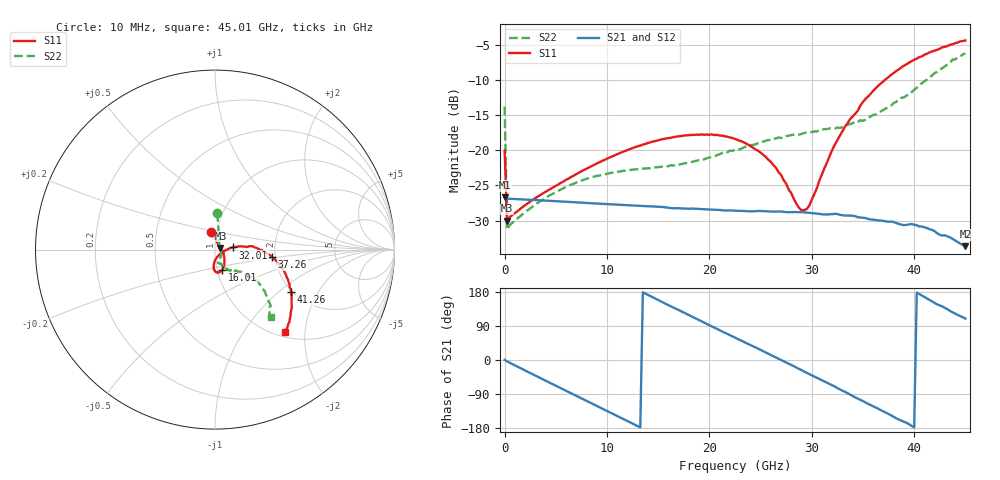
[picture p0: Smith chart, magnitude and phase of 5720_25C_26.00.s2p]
! Device:  ADRF5720
! Description: 0.5dB LSB GaAs MMIC 6-bit Digital Attenuator
! Frequency:  0.000009 -  40 GHz
! Ports:
!	RF1	= Port 1
!	RF2	= Port 2
! Vdd:  3.3 Volt
! Vss:  -3.3 Volt
! Control:  0/3.3 Volt
! State:  26.00 dB attenuation
! Data:  The device was measured using G-S-G Probes on a matrix board.
!  Data was collected using an calibrated 4 port network analyzer.
!  The reference plane for this measurement is at the launchers.
! Note:  Analog Devices supplies this data as a sample of measured data
!  for this product.  Your particular data for this product may vary.
!  Data was taken at 25 degrees C.
!  Analog Devices reserves the right to change this data at anytime.
# GHZ S DB R 45.0
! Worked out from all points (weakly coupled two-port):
!   181 points, 10 MHz to 45.01 GHz, reference 45 ohm
!   highest |S21| = -26.70 dB at 10 MHz (marker M1); lowest = -33.6 dB at 45.01 GHz (marker M2)
!   lowest |S11| = -30.0 dB at 260 MHz (marker M3), VSWR 1.07, Z = 47.8 + j0.881 ohm
!   |S11| at or under -10 dB: start of sweep to 37.16 GHz
!   |S22| runs from -31.3 to -6.2 dB; largest |S21 - S12| = 0.00012
!   S11 on the Smith chart (normalised r, x): 10 MHz: 0.94, +0.18; 16.01 GHz: 1.05, -0.25; 32.01 GHz: 1.22, +0.03; 37.26 GHz: 1.92, -0.18; 41.26 GHz: 1.97, -1.22; 45.01 GHz: 1.09, -1.57
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0.01  -20.07 103.8  -26.70 0.0  -26.71 0.0  -13.81 86.3
0.26  -30.01 16.9  -26.89 -3.8  -26.90 -3.8  -31.31 17.3
3.26  -26.59 -16.1  -27.12 -44.5  -27.11 -44.5  -27.48 -34.1
7.76  -22.81 -43.2  -27.48 -104.5  -27.48 -104.5  -24.19 -67.1
12.01  -19.97 -59.3  -27.83 -161.1  -27.82 -161.1  -22.90 -77.1
15.26  -18.49 -69.1  -28.07 154.9  -28.07 154.9  -22.36 -76.2
16.01  -18.28 -71.3  -28.18 144.7  -28.18 144.7  -22.29 -75.3
20.26  -17.76 -83.7  -28.46 88.4  -28.46 88.5  -20.94 -66.2
22.76  -18.54 -91.0  -28.63 55.7  -28.63 55.8  -19.94 -62.3
26.01  -21.66 -94.1  -28.72 13.2  -28.72 13.2  -18.57 -59.8
27.01  -23.51 -91.5  -28.72 -0.1  -28.72 -0.0  -18.26 -59.1
29.01  -28.54 -54.6  -28.82 -26.7  -28.82 -26.7  -17.69 -58.4
29.51  -28.37 -36.7  -28.88 -33.8  -28.87 -33.8  -17.47 -57.0
30.26  -26.24 -11.4  -28.98 -43.7  -28.97 -43.7  -17.32 -56.6
32.01  -19.95 6.9  -29.10 -66.5  -29.09 -66.5  -16.91 -54.1
33.26  -16.63 7.0  -29.29 -84.1  -29.29 -84.1  -16.44 -50.2
35.01  -13.14 3.4  -29.61 -108.5  -29.62 -108.5  -15.83 -46.3
37.26  -9.88 -7.5  -30.14 -139.3  -30.14 -139.2  -14.05 -39.5
37.76  -9.28 -10.1  -30.15 -146.1  -30.15 -146.0  -13.64 -38.5
41.26  -6.28 -29.1  -31.07 162.2  -31.08 162.3  -9.97 -37.7
43.76  -4.94 -42.6  -32.61 125.8  -32.62 125.8  -7.11 -45.2
45.01  -4.40 -49.8  -33.65 109.5  -33.64 109.5  -6.23 -50.6
